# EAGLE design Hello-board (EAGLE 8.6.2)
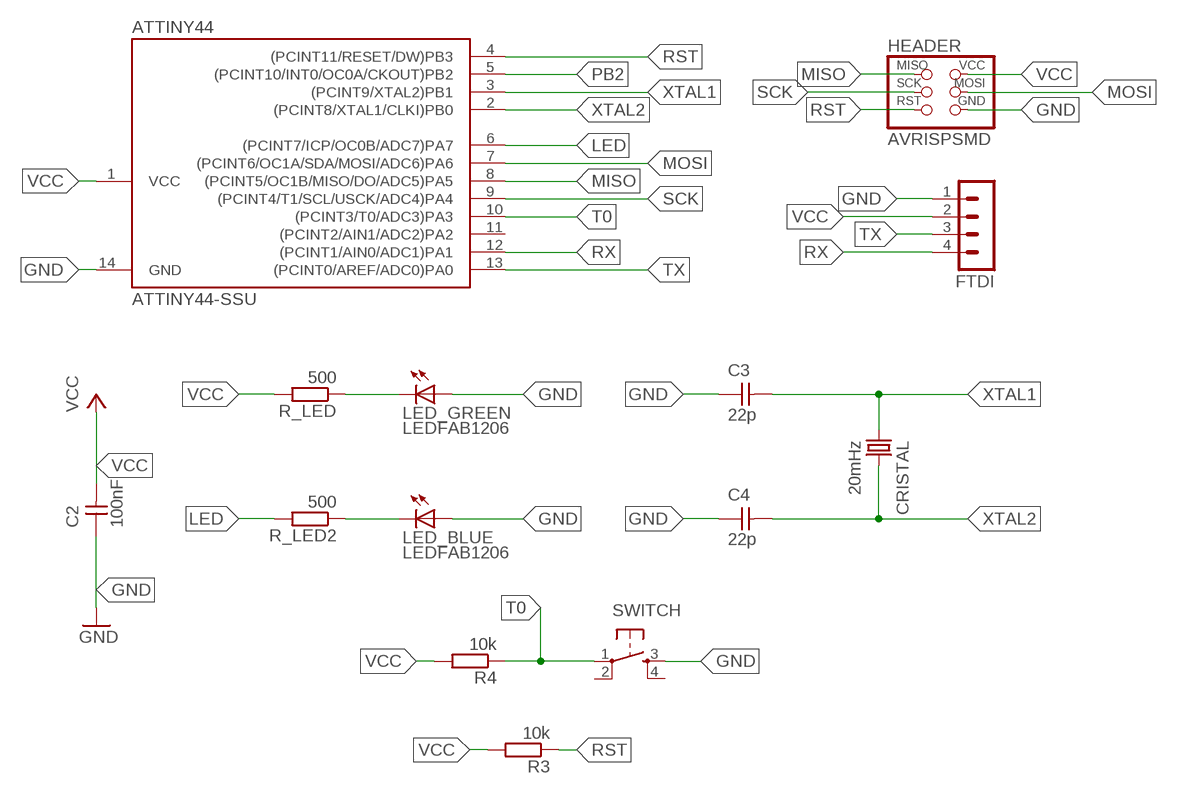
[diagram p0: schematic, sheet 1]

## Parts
ATTINY44  ATTINY44-SSU  [SOIC14]
C2  100nF  CAP-UNPOLARIZEDFAB  [C1206FAB]
C3  22p  CAP-UNPOLARIZEDFAB  [C1206FAB]
C4  22p  CAP-UNPOLARIZEDFAB  [C1206FAB]
CRISTAL  20mHz  CRYSTAL  [2-SMD-5X3MM]
FTDI  MA04-1  [MA04-1]
HEADER  AVRISPSMD  [2X03SMD]
LED_BLUE  LEDFAB1206  [LED1206FAB]
LED_GREEN  LEDFAB1206  [LED1206FAB]
R3  10k  R-EU_R1206  [R1206]
R4  10k  R-EU_R1206  [R1206]
R_LED  500  R-EU_R1206  [R1206]
R_LED2  500  R-EU_R1206  [R1206]
SWITCH  6MM_SWITCH6MM_SWITCH  [6MM_SWITCH]

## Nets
GND: ATTINY44.14(GND) C2.1 C3.1 C4.1 FTDI.1 HEADER.6(GND) LED_BLUE.1(A) LED_GREEN.1(A) SWITCH.3(S)
LED: ATTINY44.6((PCINT7/ICP/OC0B/ADC7)PA7) R_LED2.2
MISO: ATTINY44.8((PCINT5/OC1B/MISO/DO/ADC5)PA5) HEADER.1(MISO)
MOSI: ATTINY44.7((PCINT6/OC1A/SDA/MOSI/ADC6)PA6) HEADER.4(MOSI)
N$21: LED_GREEN.2(C) R_LED.1
N$22: LED_BLUE.2(C) R_LED2.1
PB2: ATTINY44.5((PCINT10/INT0/OC0A/CKOUT)PB2)
RST: ATTINY44.4((PCINT11/RESET/DW)PB3) HEADER.5(RST) R3.1
RX: ATTINY44.12((PCINT1/AIN0/ADC1)PA1) FTDI.4
SCK: ATTINY44.9((PCINT4/T1/SCL/USCK/ADC4)PA4) HEADER.3(SCK)
T0: ATTINY44.10((PCINT3/T0/ADC3)PA3) R4.1 SWITCH.1(P)
TX: ATTINY44.13((PCINT0/AREF/ADC0)PA0) FTDI.3
VCC: ATTINY44.1(VCC) C2.2 FTDI.2 HEADER.2(VCC) R3.2 R4.2 R_LED.2
XTAL1: ATTINY44.3((PCINT9/XTAL2)PB1) C3.2 CRISTAL.P$1
XTAL2: ATTINY44.2((PCINT8/XTAL1/CLKI)PB0) C4.2 CRISTAL.P$2
Unconnected: ATTINY44.11((PCINT2/AIN1/ADC2)PA2) SWITCH.2(P1) SWITCH.4(S1)

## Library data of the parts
ATTINY44 = fab:ATTINY44
C2-C4 = fab:CAP-UNPOLARIZED
CRISTAL = fab:CRYSTAL
FTDI = con-lstb:MA04-1: PIN HEADER; OC_FARNELL: unknown; OC_NEWARK: unknown
HEADER = fab:AVRISP
LED_BLUE LED_GREEN = fab:LED: LED
R3 R4 R_LED R_LED2 = resistor:R-EU_: RESISTOR, European symbol
SWITCH = fab:6MM_SWITCH: OMRON SWITCH

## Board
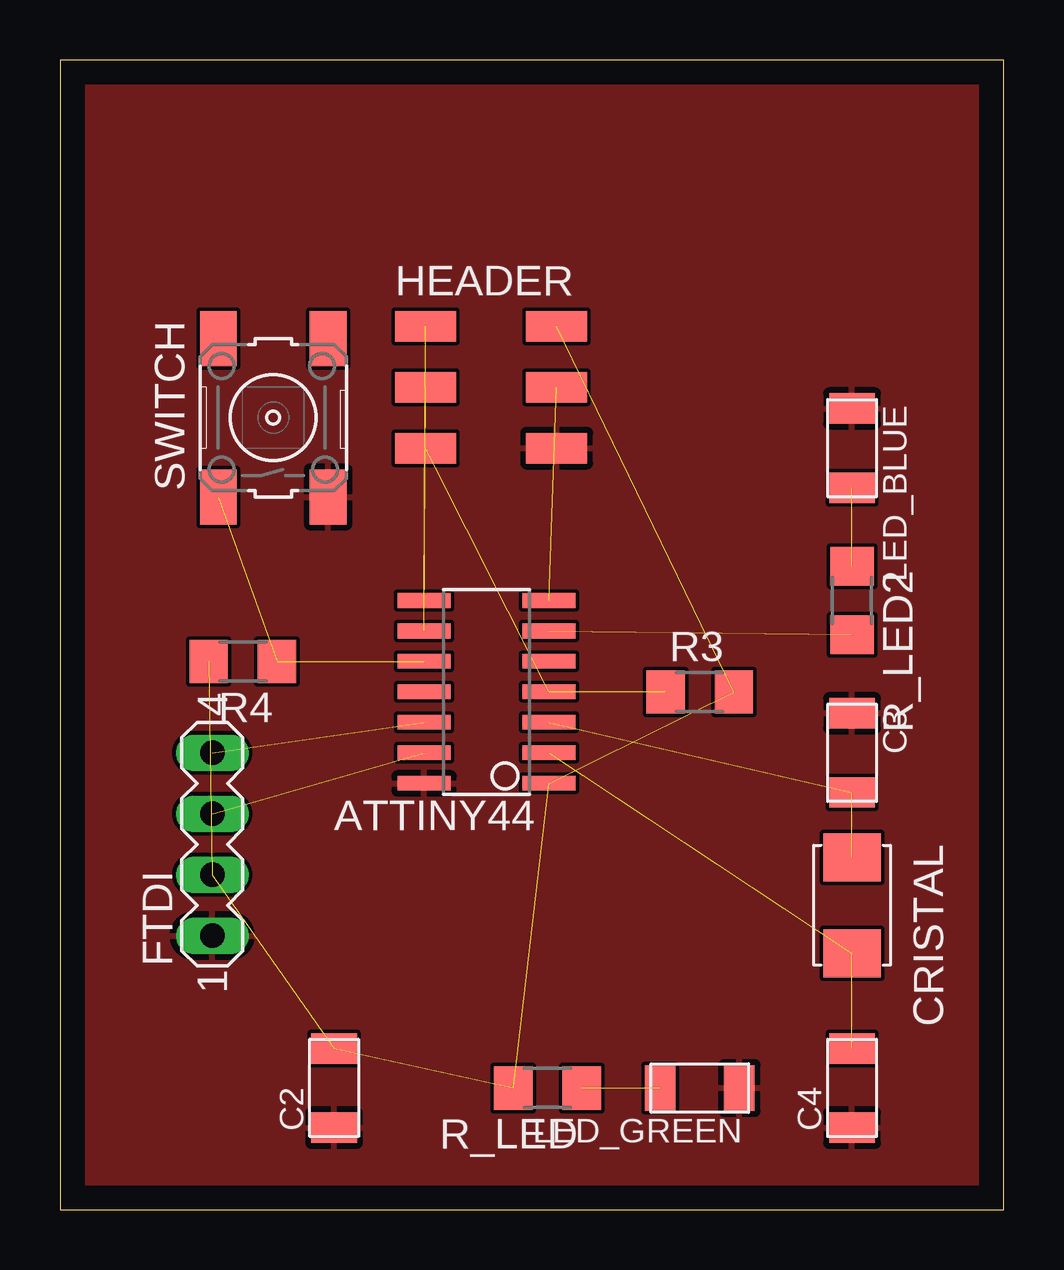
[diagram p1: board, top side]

Size 39.35 x 47.93 mm. Coordinates in mm from the lower left corner, seen from the top.
Outline: 0,0 39.35,0 39.35,47.93 0,47.93 0,0
Copper layers (1*16): Top 0.035mm / dielectric 1.5mm / Bottom 0.035mm
Design rules "default": minimum track width 6mil, minimum drill 0.35mm, track to track 6mil, track to pad 6mil, pad to pad 6mil, via to via 6mil, smd to smd 6mil, copper to edge 40mil, drill to drill 6mil, minimum pad ring 10mil, minimum via ring 8mil, stop-mask expansion 4mil, vias tented up to drill 0mil, thermal gap 10mil

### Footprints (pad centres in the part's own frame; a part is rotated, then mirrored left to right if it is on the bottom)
SOIC14 = smd 0.61 x 2.21: 1 -3.81,-2.603; 2 -2.54,-2.603; 3 -1.27,-2.603; 4 0,-2.603; 5 1.27,-2.603; 6 2.54,-2.603; 7 3.81,-2.603; 8 3.81,2.603; 9 2.54,2.603; 10 1.27,2.603; 11 0,2.603; 12 -1.27,2.603; 13 -2.54,2.603; 14 -3.81,2.603
C1206FAB = smd 1.27 x 1.905: 1 -1.651,0; 2 1.651,0
2-SMD-5X3MM = smd 2 x 2.4: P$1 -2,0; P$2 2,0
MA04-1 = drill 1.016 long: 1 -3.81,0; 2 -1.27,0; 3 1.27,0; 4 3.81,0
2X03SMD = smd 2.54 x 1.27: 1 -2.54,2.54; 2 2.92,2.54; 3 -2.54,0; 4 2.92,0; 5 -2.54,-2.54; 6 2.92,-2.54
LED1206FAB = smd 1.27 x 1.905: 1 -1.651,0; 2 1.651,0
R1206 = smd 1.6 x 1.803: 1 -1.422,0; 2 1.422,0
6MM_SWITCH = smd 2.286 x 1.524: 1 -3.302,2.286; 2 3.302,2.286; 3 -3.302,-2.286; 4 3.302,-2.286

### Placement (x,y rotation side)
ATTINY44  17.78,21.59 90 top
C2  11.43,5.08 90 top
C3  33.02,19.05 270 top
C4  33.02,5.08 90 top
CRISTAL  33.02,12.7 270 top
FTDI  6.35,15.24 90 top
HEADER  17.78,34.29 0 top
LED_BLUE  33.02,31.75 270 top
LED_GREEN  26.67,5.08 180 top
R3  26.67,21.59 0 top
R4  7.62,22.86 180 top
R_LED  20.32,5.08 180 top
R_LED2  33.02,25.4 270 top
SWITCH  8.89,33.02 90 top

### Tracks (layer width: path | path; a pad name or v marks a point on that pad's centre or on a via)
GND
  pour Top: -7.62,52.07 -7.62,-3.81 46.99,-3.81 46.99,52.07
LED  (1 unrouted)
MISO  (1 unrouted)
MOSI  (1 unrouted)
N$21  (1 unrouted)
N$22  (1 unrouted)
RST  (2 unrouted)
RX  (1 unrouted)
SCK  (1 unrouted)
T0  (2 unrouted)
TX  (1 unrouted)
VCC  (6 unrouted)
XTAL1  (2 unrouted)
XTAL2  (2 unrouted)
